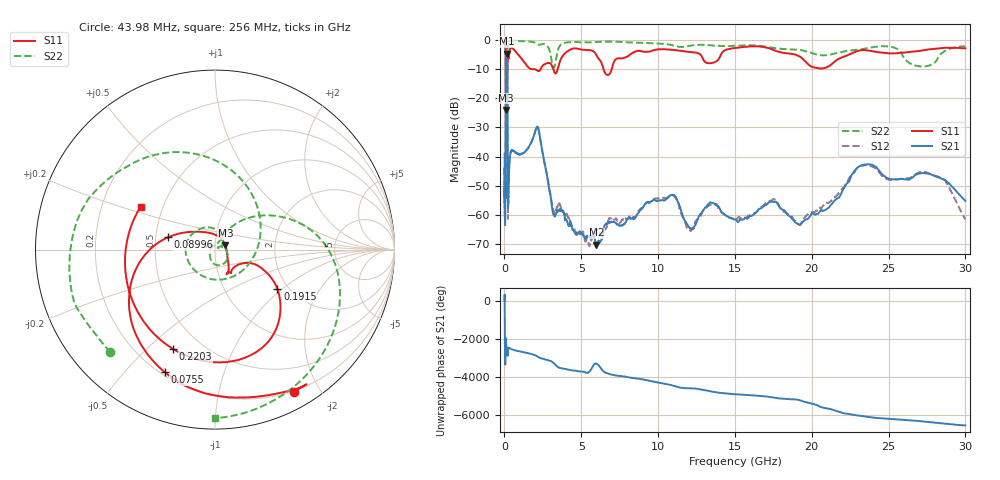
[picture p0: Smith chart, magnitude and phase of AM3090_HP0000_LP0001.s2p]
! Date/Time: Thu, Feb 28, 2019 1:52 PM
! Network Analyzer: Agilent Technologies E8364B Rev: A.07.50.67
! Sweep from 0.010 to 30.000 GHz, 1601 Points, Sweep Type: LOG
! Power Supply: 5.022 V, 0.002 A
# Hz S DB R 50
!freq MagS11 AngS11 MagS21 AngS21 MagS12 AngS12 MagS22 AngS22
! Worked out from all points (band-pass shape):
!   1601 points, 10 MHz to 30 GHz, reference 50 ohm
!   highest |S21| = -4.63 dB at 134.2 MHz (marker M1); lowest = -70.2 dB at 5.989 GHz (marker M2)
!   |S21| within 3 dB of the highest: 97.86 MHz to 177.4 MHz (79.57 MHz wide, 57.8 % of centre)
!   lowest |S11| = -24.0 dB at 97.46 MHz (marker M3), VSWR 1.13, Z = 56.1 + j2.81 ohm
!   |S11| at or under -10 dB: 1.979 GHz to 2.355 GHz (376.1 MHz wide, 17.4 % of centre); 3.18 GHz to 3.465 GHz (285.5 MHz wide, 8.59 % of centre); 6.454 GHz to 6.981 GHz (526.9 MHz wide, 7.84 % of centre)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
!   |S22| runs from -35.1 to -0.1 dB; largest |S21 - S12| = 0.017
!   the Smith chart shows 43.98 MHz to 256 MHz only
!   S11 on the Smith chart (normalised r, x): 43.98 MHz: 0.19, -1.69; 75.5 MHz: 0.22, -0.65; 89.96 MHz: 0.58, +0.09; 191.5 MHz: 1.75, -0.92; 220.3 MHz: 0.35, -0.60; 256 MHz: 0.37, +0.23
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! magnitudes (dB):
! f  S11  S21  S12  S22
! 10 MHz  -0.2  -38.9  -44.0  -0.6
! 38.04 MHz  -0.5  -62.4  -62.3  -1.4
! 43.98 MHz  -0.8  -57.5  -59.1  -1.8
! 75.5 MHz  -2.6  -43.6  -42.5  -5.0
! 89.96 MHz  -11.4  -14.1  -14.2  -15.5
! 97.46 MHz  -24.0  -7.8  -7.8  -16.0
! 134.2 MHz  -16.5  -4.6  -4.6  -28.6
! 144.7 MHz  -16.0  -4.7  -4.7  -21.5
! 170.7 MHz  -15.3  -6.4  -6.3  -33.2
! 191.5 MHz  -7.7  -16.4  -16.4  -11.1
! 220.3 MHz  -4.4  -57.1  -59.3  -1.5
! 256 MHz  -6.4  -53.9  -54.2  -0.5
! 550.5 MHz  -3.0  -38.1  -37.9  -0.2
! 2.084 GHz  -10.3  -30.0  -30.1  -1.2
! 3.204 GHz  -10.4  -60.0  -58.9  -9.6
! 5.989 GHz  -5.2  -70.2  -65.4  -0.7
! 7.926 GHz  -5.9  -62.1  -61.6  -0.8
! 10.76 GHz  -3.3  -53.5  -53.8  -1.6
! 12.07 GHz  -4.1  -64.4  -65.3  -2.0
! 19.51 GHz  -6.9  -61.9  -61.2  -3.7
! 23.48 GHz  -3.5  -42.7  -42.9  -2.9
! 30 GHz  -2.8  -55.2  -61.6  -2.2
